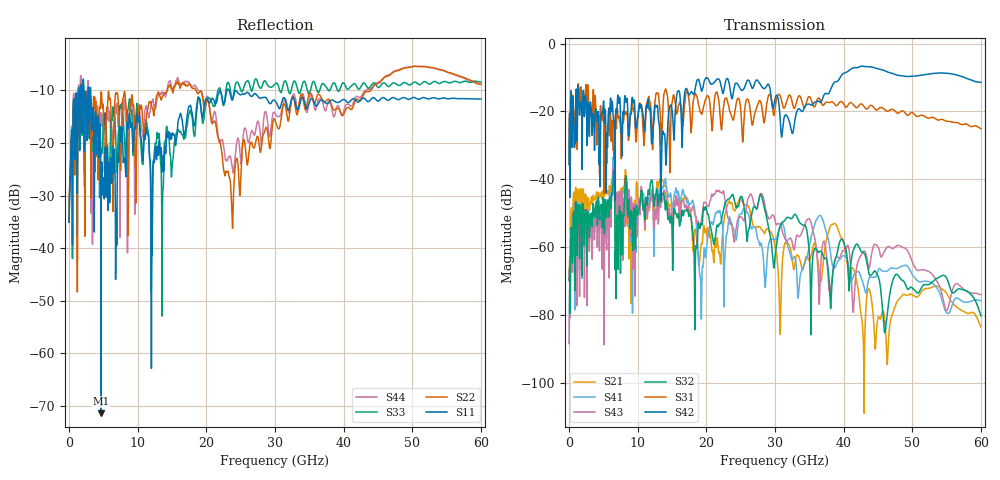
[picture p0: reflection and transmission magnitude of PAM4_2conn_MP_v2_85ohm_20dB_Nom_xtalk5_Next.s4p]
! Info: Touchstone file created by Circ.  Input file=FAB50GbE_2conn_Midplane_Examax_Topo2_v2_85ohm_20dB_Nom.circ
# Hz S RI R 50
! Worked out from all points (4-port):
!   6000 points, 10 MHz to 60 GHz, reference 50 ohm
!   strongest paths, dB at 10 MHz, 15.01 GHz, 30.01 GHz, 45.01 GHz, 60 GHz:
!     S42: -35.6, -19.6, -16.3, -7.5, -11.4
!     S31: -35.8, -17.4, -19.3, -19.4, -25.1
!     S32: -69.9, -54.9, -62.9, -68.6, -80.2
!     S43: -88.5, -52.1, -52.1, -59.9, -74.1
!     S41: -88.2, -47.5, -57.8, -67.0, -75.8
!     S21: -69.5, -51.0, -59.8, -80.9, -83.5
!   lowest |S11| = -71.4 dB at 4.66 GHz (marker M1), VSWR 1.00, Z = 50 - j0.0118 ohm
!   |S11| at or under -10 dB: start of sweep to 1.333 GHz; 3.153 GHz to 23.01 GHz (19.85 GHz wide, 152 % of centre); 23.33 GHz to end of sweep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
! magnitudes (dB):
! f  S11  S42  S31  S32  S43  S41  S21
! 10 MHz  -35.1  -35.6  -35.8  -69.9  -88.5  -88.2  -69.5
! 4.66 GHz  -71.4  -21.5  -20.4  -47.5  -50.7  -48.8  -44.3
! 23.76 GHz  -11.8  -16.3  -21.9  -44.5  -54.3  -53.6  -47.2
! 30.72 GHz  -13.4  -21.0  -15.3  -54.2  -53.2  -53.8  -83.4
! 38.62 GHz  -12.0  -11.5  -17.7  -65.0  -65.0  -66.3  -53.0
! 42.79 GHz  -11.5  -6.7  -18.1  -61.5  -61.5  -70.3  -84.2
! 60 GHz  -11.6  -11.4  -25.1  -80.2  -74.1  -75.8  -83.5
